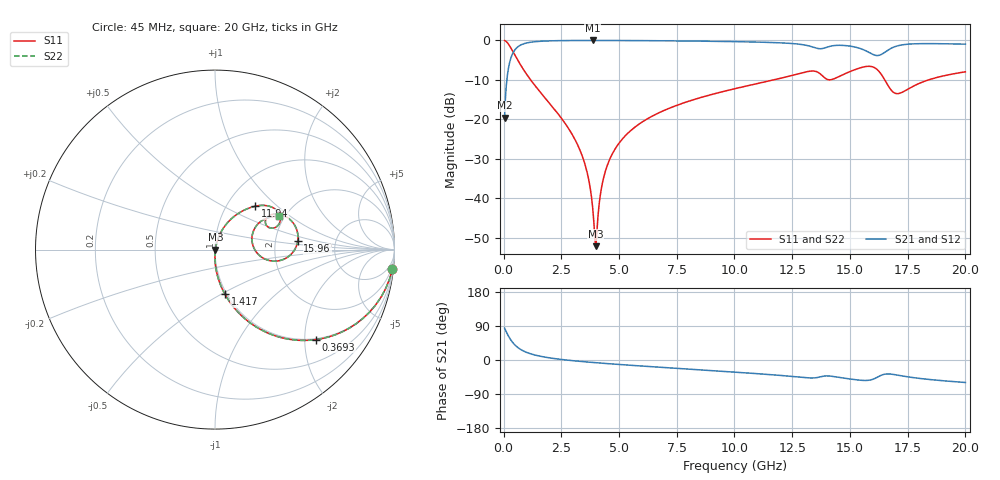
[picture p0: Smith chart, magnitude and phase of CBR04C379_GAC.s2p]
! S-parameter model data by Modelithics Inc.  support@modelithics.com 813-866-6335  Tampa FL USA
! S-Parameter data specifications:
! Substrate: 20-mil Rogers 4350B, substrate thickness, H=0.508mm, Dielectric constant, Er=3.75
! PCB Mounting Pad Footprint: Pad width, PadW=0.52mm , Pad length, PadL=0.52mm , Pad gap, PadG (edge-to-edge)=0.28mm , Reference planes=1.32mm apart
#  GHz  S  MA  R 50
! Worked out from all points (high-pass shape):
!   801 points, 45 MHz to 20 GHz, reference 50 ohm
!   highest |S21| = -0.02 dB at 3.861 GHz (marker M1); lowest = -19.6 dB at 45 MHz (marker M2)
!   |S21| within 3 dB of the highest: 421.8 MHz to 15.82 GHz (15.39 GHz wide, 190 % of centre); 16.51 GHz to end of sweep
!   lowest |S11| = -52.2 dB at 3.986 GHz (marker M3), VSWR 1.00, Z = 50.2 - j0.0449 ohm
!   |S11| at or under -10 dB: 1.171 GHz to 11.71 GHz (10.54 GHz wide, 164 % of centre); 16.51 GHz to 18.41 GHz (1.908 GHz wide, 10.9 % of centre)
!   |S22| runs from -52.2 to 0.0 dB; largest |S21 - S12| = 0
!   S11 on the Smith chart (normalised r, x): 45 MHz: 1, -19; 369.3 MHz: 0.98, -2.26; 1.417 GHz: 0.98, -0.52; 11.94 GHz: 1.35, +0.73; 15.96 GHz: 2.68, +0.33; 20 GHz: 1.86, +0.82
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0.045  0.9945 -6.1  0.1048 83.9  0.1048 83.9  0.9945 -6.1
0.219606  0.8886 -27.7  0.4583 62.3  0.4583 62.3  0.8886 -27.7
0.369269  0.7534 -41.7  0.6569 48.2  0.6569 48.2  0.7534 -41.7
0.768369  0.4717 -63.1  0.8807 26.8  0.8807 26.8  0.4717 -63.1
1.416906  0.2548 -77.4  0.9655 12.2  0.9655 12.2  0.2548 -77.4
2.738925  0.08254 -88.8  0.9945 -0.2  0.9945 -0.2  0.08254 -88.8
3.387462  0.03548 -90.4  0.997 -4.0  0.997 -4.0  0.03548 -90.4
3.686787  0.0172 -87.7  0.9974 -5.6  0.9974 -5.6  0.0172 -87.7
3.861394  0.007432 -77.5  0.9974 -6.5  0.9974 -6.5  0.007432 -77.5
3.986112  0.002468 -10.4  0.9974 -7.1  0.9974 -7.1  0.002468 -10.4
4.310381  0.01705 72.7  0.9972 -8.7  0.9972 -8.7  0.01705 72.7
4.734425  0.0376 75.3  0.9964 -10.6  0.9964 -10.6  0.0376 75.3
6.704981  0.12 69.5  0.9892 -18.9  0.9892 -18.9  0.12 69.5
10.0225  0.2445 56.7  0.9638 -32.0  0.9638 -32.0  0.2445 56.7
11.94317  0.3281 47.3  0.9317 -40.5  0.9317 -40.5  0.3281 47.3
13.36496  0.4092 30.2  0.8282 -47.4  0.8282 -47.4  0.4092 30.2
14.16316  0.3168 27.1  0.8445 -42.6  0.8445 -42.6  0.3168 27.1
15.18586  0.4224 27.1  0.8271 -51.6  0.8271 -51.6  0.4224 27.1
15.95911  0.4637 6.0  0.6711 -51.6  0.6711 -51.6  0.4637 6.0
16.68248  0.2585 -8.7  0.764 -36.8  0.764 -36.8  0.2585 -8.7
17.13147  0.2126 14.4  0.8622 -40.7  0.8622 -40.7  0.2126 14.4
20  0.3996 27.6  0.8952 -59.4  0.8952 -59.4  0.3996 27.6
